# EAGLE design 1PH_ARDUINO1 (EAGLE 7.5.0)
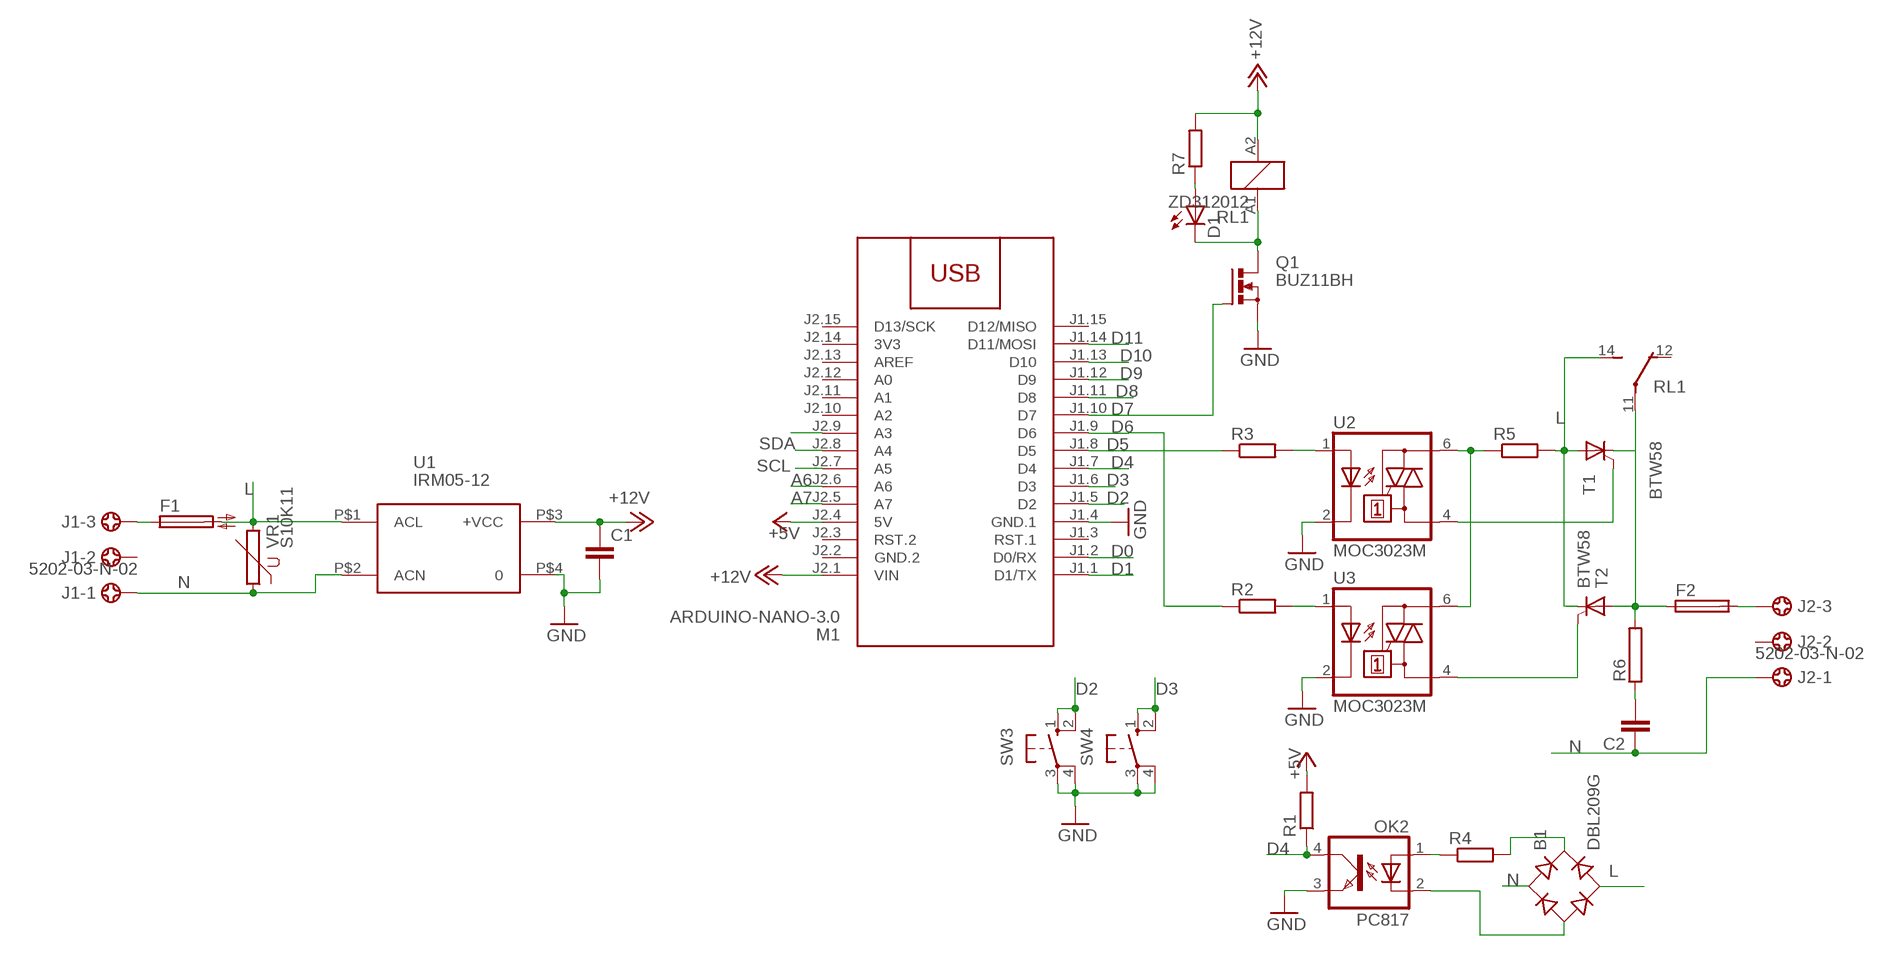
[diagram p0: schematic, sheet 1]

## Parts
B1  DBL209G  [DB]
C1  C-EUC1206  [C1206]
C2  C-EU150-084X183  [C150-084X183]
D1  LED5MM  [LED5MM]
F1  SH22,5A  [SH22,5A]
F2  SH22,5A  [SH22,5A]
J1  5202-03-N-02  [5202-03-N-02]
J2  5202-03-N-02  [5202-03-N-02]
M1  ARDUINO-NANO-3.0  [ARDUINO-NANO-3.0]
OK2  PC817  [DIL04]
Q1  BUZ11BH  [TO220BH]
R1  R-EU_R1206  [R1206]
R2  R-EU_R1206  [R1206]
R3  R-EU_R1206  [R1206]
R4  R-EU_R1206  [R1206]
R5  R-EU_R1206  [R1206]
R6  RAC07  [AC07]
R7  R-EU_R1206  [R1206]
RL1  ZD312012  [ZD1]
SW3  10-XX  [B3F-10XX]
SW4  10-XX  [B3F-10XX]
T1  BTW58  [TO220CS]
T2  BTW58  [TO220CS]
U1  IRM05-12  [IRM05-12]
U2  MOC3023M  [DIL06]
U3  MOC3023M  [DIL06]
VR1  S10K11  [S10K11]

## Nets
+5V: M1.J2.4(5V) R1.2
+12V: C1.1 M1.J2.1(VIN) R7.2 RL1.A2 U1.P$3(+VCC)
A3: M1.J2.9(A3)
A6: M1.J2.6(A6)
A7: M1.J2.5(A7)
D0: M1.J1.2(D0/RX)
D1: M1.J1.1(D1/TX)
D2: M1.J1.5(D2) SW3.1(S) SW3.2(S1)
D3: M1.J1.6(D3) SW4.1(S) SW4.2(S1)
D4: M1.J1.7(D4) OK2.4(COL) R1.1
D5: M1.J1.8(D5) R3.1
D6: M1.J1.9(D6) R2.1
D7: M1.J1.10(D7) Q1.G
D8: M1.J1.11(D8)
D9: M1.J1.12(D9)
D10: M1.J1.13(D10)
D11: M1.J1.14(D11/MOSI)
GND: C1.2 M1.J1.4(GND.1) OK2.3(EMIT) Q1.S SW3.3(P) SW3.4(P1) SW4.3(P) SW4.4(P1) U1.P$4 U2.2(C) U3.2(C)
L: B1.AC2 F1.2 R5.2 RL1.14(2:S) T1.A T2.C U1.P$1(ACL) VR1.2
N: B1.AC1 C2.1 J1.1 J2.1 U1.P$2(ACN) VR1.1
N$1: T2.G U3.4(A1)
N$2: R3.2 U2.1(A)
N$3: R2.2 U3.1(A)
N$4: R5.1 U2.6(A2) U3.6(A2)
N$5: B1.+ R4.2
N$6: OK2.1(A) R4.1
N$7: B1.- OK2.2(C)
N$8: F1.1 J1.3
N$9: T1.G U2.4(A1)
N$11: F2.1 R6.2 RL1.11(2:P) T1.C T2.A
N$12: D1.K(C) Q1.D RL1.A1
N$13: C2.2 R6.1
N$14: F2.2 J2.3
N$17: D1.A R7.1
SCL: M1.J2.7(A5)
SDA: M1.J2.8(A4)
Unconnected: J1.2 J2.2 M1.J1.3(RST.1) M1.J1.15(D12/MISO) M1.J2.3(RST.2) M1.J2.10(A2) M1.J2.11(A1) M1.J2.12(A0) M1.J2.13(AREF) M1.J2.15(D13/SCK) RL1.12(2:O)

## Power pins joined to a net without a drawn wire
3V3: M1.J2.14(3V3)
GND.2: M1.J2.2(GND.2)

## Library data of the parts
B1 = rectifier:DB?*G: Single Phase 1.0 AMP Glass Passivated Bridge Rectifier Taiwan Semiconductor Co.,Ltd. - TSC Source: http://www.taiwansemi.com/TSCbig5/ezcatfiles/cust/img/img/db101g.pdf http://www.ts.com.tw/db/pictures/modules/PDT/PDT060207001/DBLS201G.pdf
C1 C2 = rcl:C-EU: CAPACITOR, European symbol
D1 = led:LED: LED
F1 F2 = fuse:SH22,5A: FUSE HOLDER; MPN: 0031.7701.11; OC_FARNELL: unknown; OC_NEWARK: 04F1224
J1 J2 = con-ebyelectro:5202-03-N-02: Barrier Blocks Sreies 5202 Source: http://www.ebyelectro.com/PDF/5202-XX-N-02.pdf; OC_FARNELL: unknown; OC_NEWARK: unknown
M1 = diy-modules:ARDUINO-NANO-3.0: Arduino Nano 3.0 and compatible devices More details available here: https://www.arduino.cc/en/Main/ArduinoBoardNano Click here to find device on ebay.com
OK2 = optocoupler:PC817: SHARP OPTO COUPLER; MPN: PC817X4J000F; OC_FARNELL: 9707727; OC_NEWARK: 97K7059
Q1 = transistor-power:BUZ11: N-CHANNEL MOS FET
R1-R5 R7 = rcl:R-EU_: RESISTOR, European symbol
R6 = resistor-power:R: Power Resitor; OC_FARNELL: unknown; OC_NEWARK: unknown
RL1 = relay:ZD?1*: Power Relay SCHRACK 1 pole 30 A Source: http://www.schrack.com/.. 5848.pdf; OC_FARNELL: unknown; OC_NEWARK: unknown
SW3 SW4 = switch-omron:10-XX: OMRON SWITCH; MPN: B3F-1000; OC_FARNELL: 176432; OC_NEWARK: 36M3542
T1 T2 = triac:BTW58: THYRISTOR
U1 = acdc:IRM05-12
U2 U3 = optocoupler:MOC30*M: RANDOM-PHASE OPTOISOLATORS TRIAC DRIVER OUTPUT Source: http://www.fairchildsemi.com MOC3020-M.pdf; MF: FAIRCHILD SEMICONDUCTOR; MPN: MOC3023-M; OC_FARNELL: 1021367; OC_NEWARK: 72K8896
VR1 = varistor:S10K11: VARISTOR

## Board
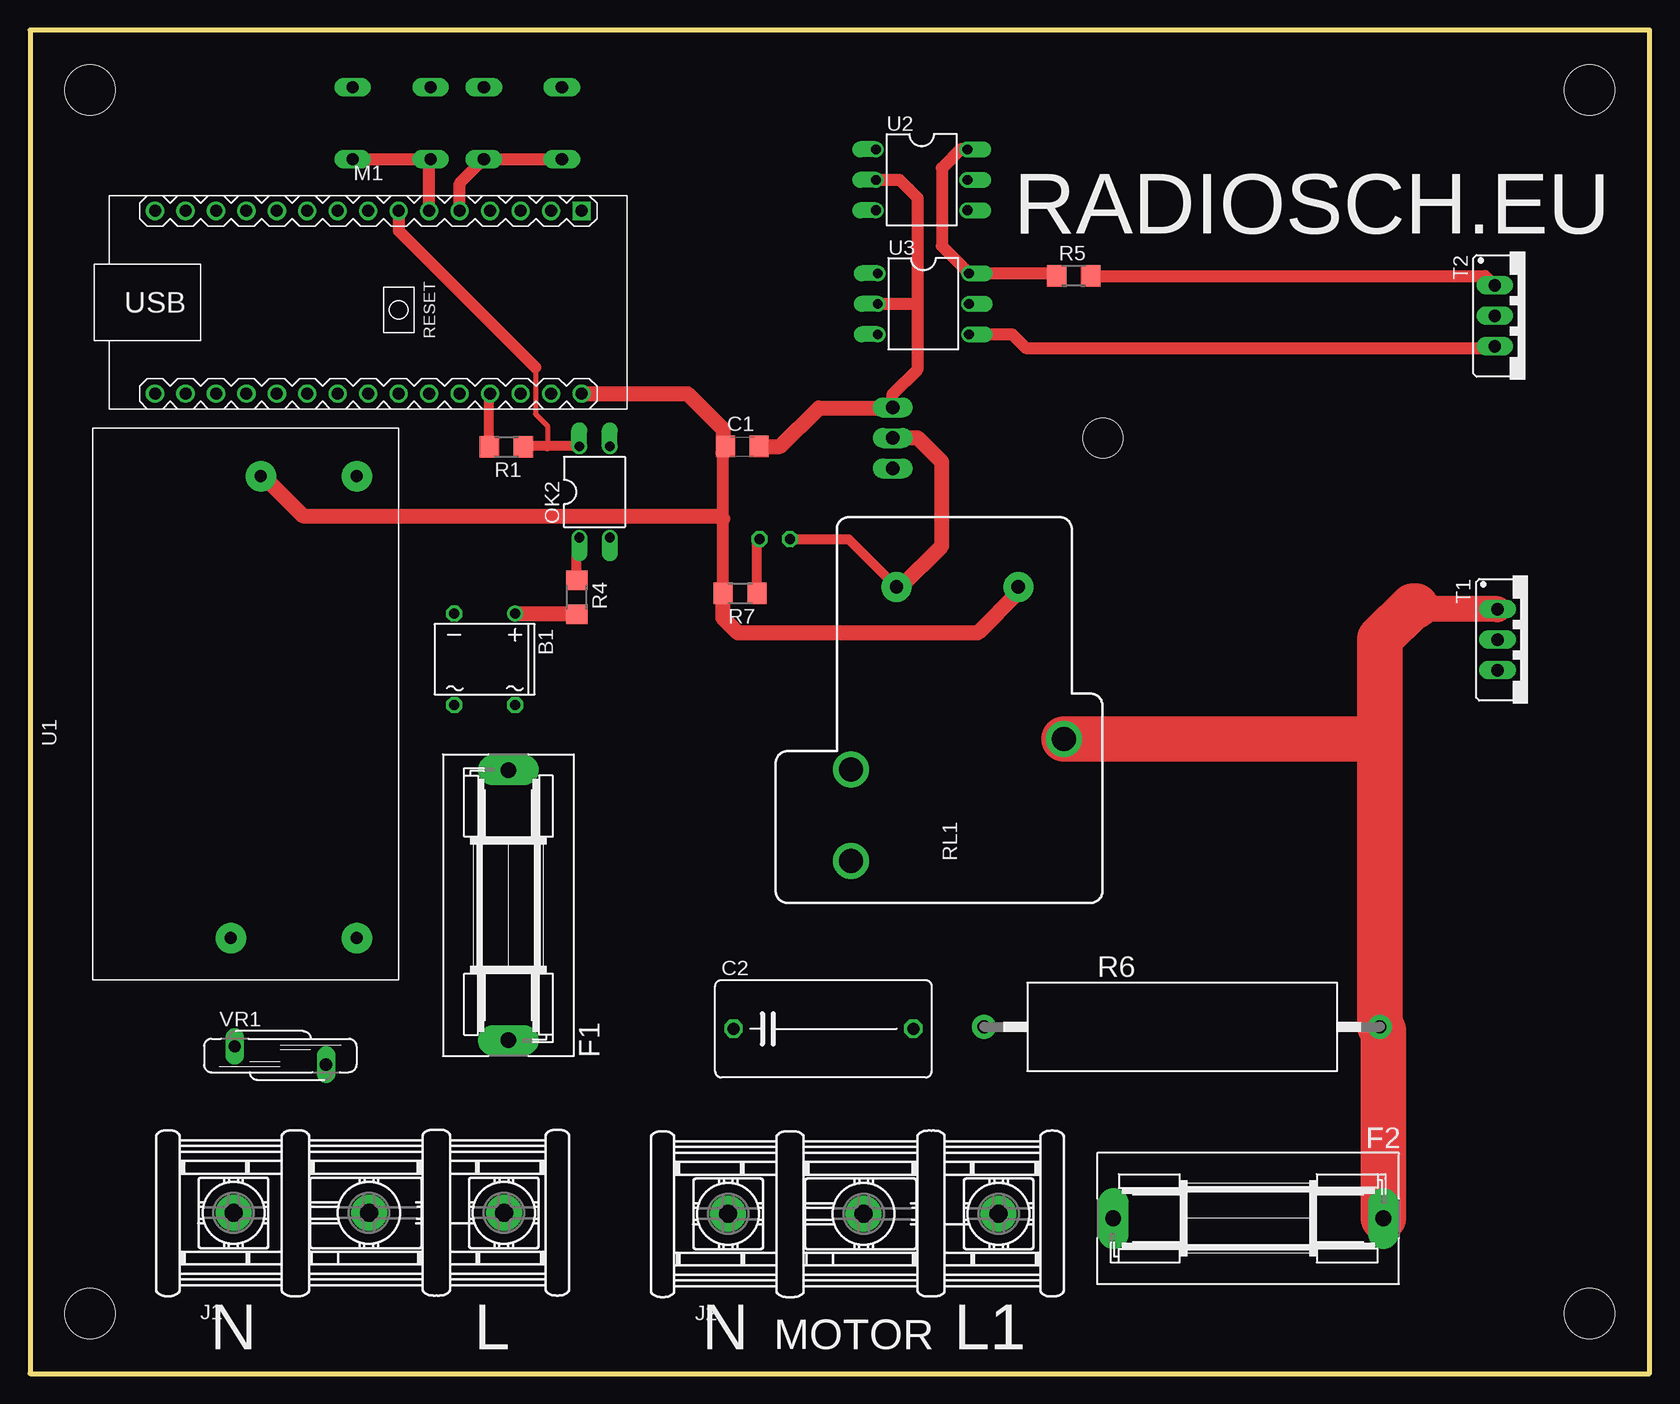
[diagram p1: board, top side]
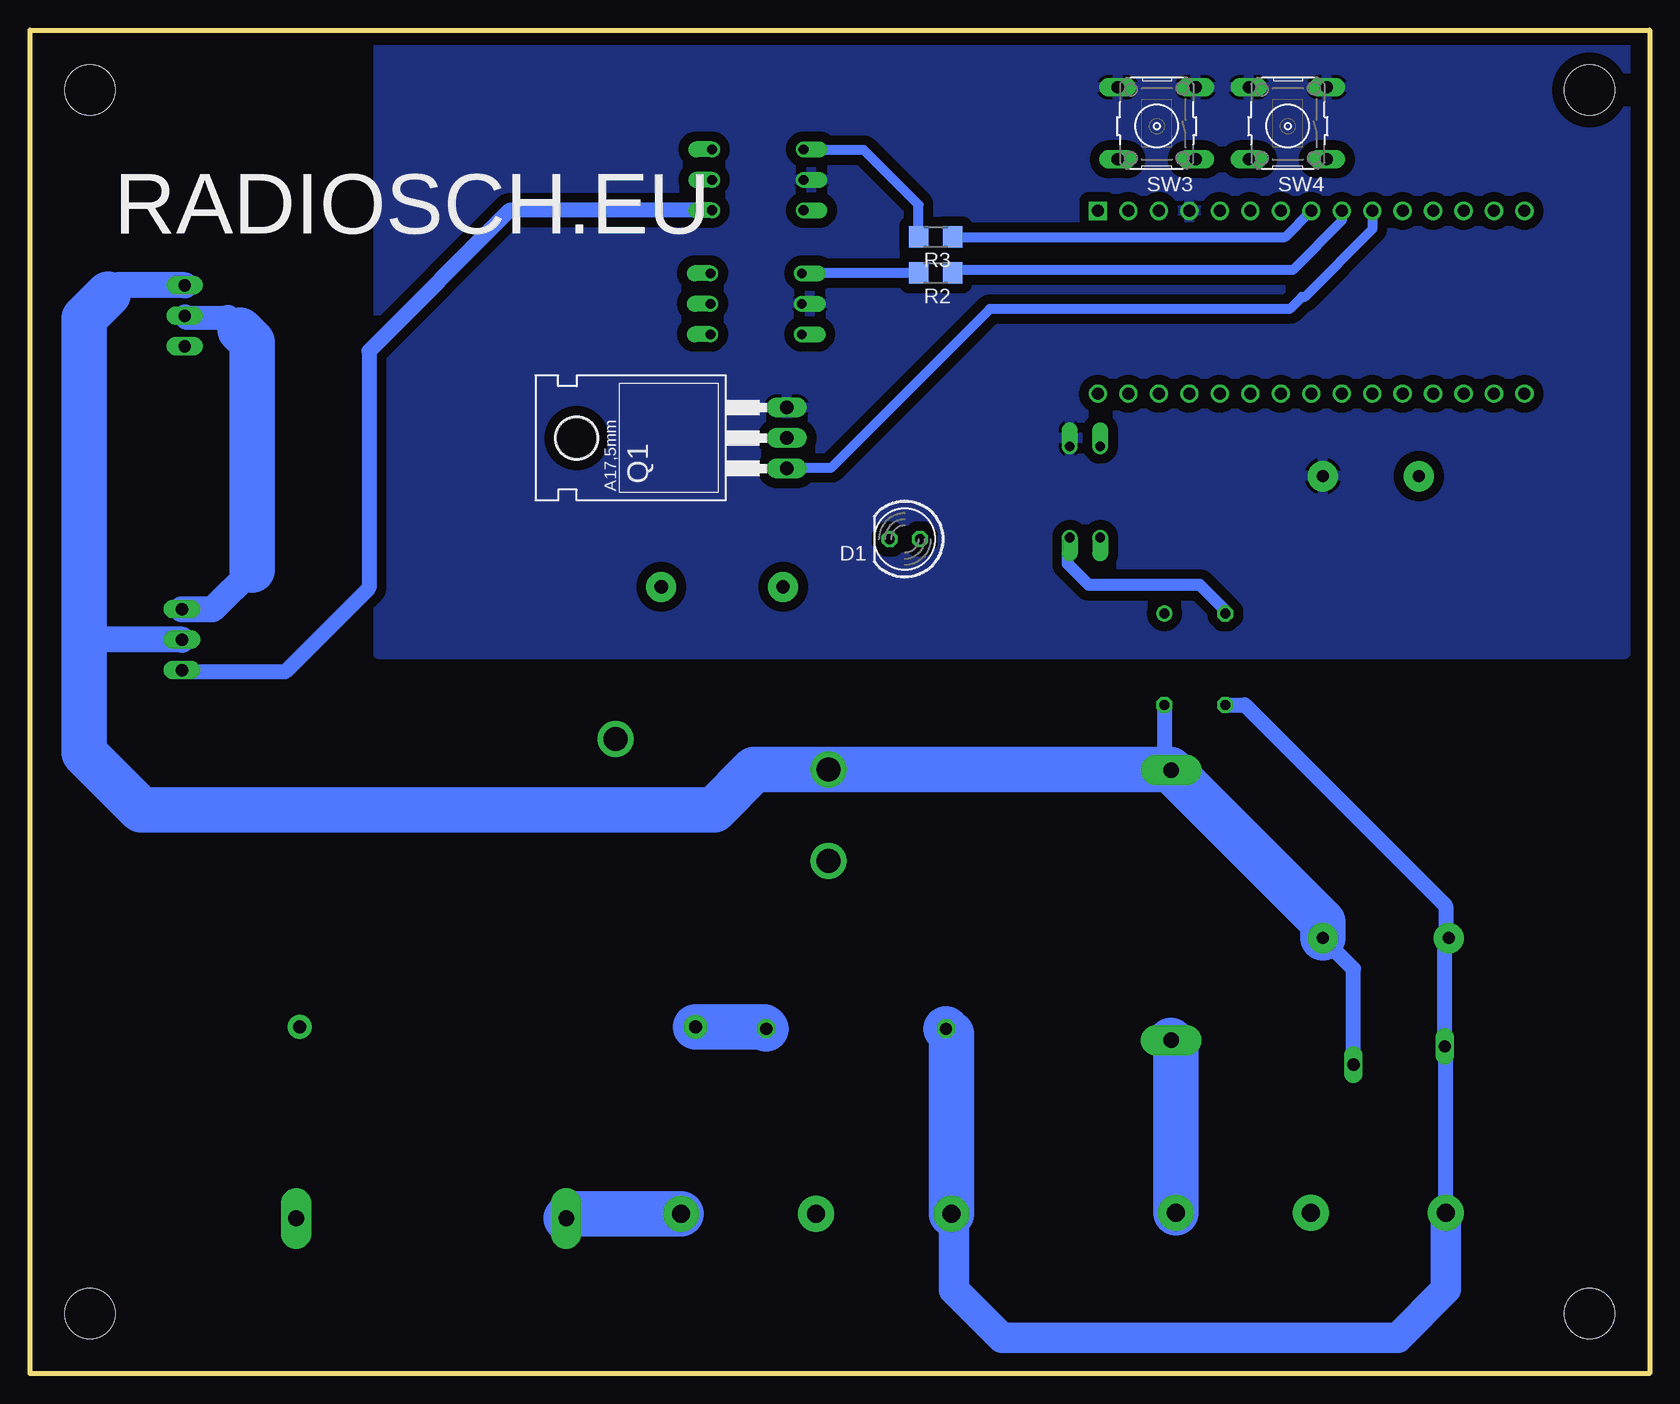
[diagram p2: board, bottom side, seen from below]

Size 135 x 112 mm. Coordinates in mm from the lower left corner, seen from the top.
Outline: 0,0 135,0 135,112 0,112 0,0
Copper layers (1*16): Top 0.035mm / dielectric 1.5mm / Bottom 0.035mm
Design rules "default": minimum track width 10mil, minimum drill 24mil, track to track 8mil, track to pad 8mil, pad to pad 8mil, via to via 8mil, smd to smd 8mil, copper to edge 40mil, drill to drill 8mil, minimum pad ring 10mil, minimum via ring 8mil, stop-mask expansion 4mil, vias tented up to drill 0mil, thermal gap 10mil
Holes 4.2 mm at 5,107 130,107 130,5 5,5

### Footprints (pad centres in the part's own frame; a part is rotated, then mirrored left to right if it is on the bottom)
DB = drill 0.813: + -2.54,-3.81 | drill 0.813 octagon: - 2.54,-3.81; AC1 2.54,3.81; AC2 -2.54,3.81
C1206 = smd 1.6 x 1.8: 1 -1.4,0; 2 1.4,0
C150-084X183 = drill 1.016 octagon: 1 -7.493,0; 2 7.493,0
LED5MM = drill 0.813 octagon: A -1.27,0; K 1.27,0
SH22,5A = drill 1.321 pad 2.54 long: 1 -11.252,0; 2 11.252,0
5202-03-N-02 = drill 1.5 pad 3: 1 -9.29,0; 2 2,0; 3 13.25,0
ARDUINO-NANO-3.0 = drill 1 square: J1.1 17.78,7.62 | drill 1: J1.2 15.24,7.62; J1.3 12.7,7.62; J1.4 10.16,7.62; J1.5 7.62,7.62; J1.6 5.08,7.62; J1.7 2.54,7.62; J1.8 0,7.62; J1.9 -2.54,7.62; J1.10 -5.08,7.62; J1.11 -7.62,7.62; J1.12 -10.16,7.62; J1.13 -12.7,7.62; J1.14 -15.24,7.62; J1.15 -17.78,7.62; J2.1 17.78,-7.62; J2.2 15.24,-7.62; J2.3 12.7,-7.62; J2.4 10.16,-7.62; J2.5 7.62,-7.62; J2.6 5.08,-7.62; J2.7 2.54,-7.62; J2.8 0,-7.62; J2.9 -2.54,-7.62; J2.10 -5.08,-7.62; J2.11 -7.62,-7.62; J2.12 -10.16,-7.62; J2.13 -12.7,-7.62; J2.14 -15.24,-7.62; J2.15 -17.78,-7.62
DIL04 = drill 0.813 offset: 1 -1.27,-3.81; 2 1.27,-3.81; 3 1.27,3.81; 4 -1.27,3.81
TO220BH = drill 1.118 long: D 0,-6.35; G -2.54,-6.35; S 2.54,-6.35 | hole 3.302: 0,11.176
R1206 = smd 1.6 x 1.803: 1 -1.422,0; 2 1.422,0
AC07 = drill 1.1 pad 2: 1 -16.5,0; 2 16.5,0
ZD1 = drill 2 pad 2.5: 11 -2.54,-8.88; 12 -12.7,8.88; 14 -5.08,8.88 | drill 1.1 pad 2.5: A1 10.16,5.08; A2 10.16,-5.08
B3F-10XX = drill 1.016 long: 1 -3.251,2.761; 2 3.251,2.761; 3 -3.251,-3.261; 4 3.251,-3.261
TO220CS = drill 1.016 long: A 0,-2.54; C -2.54,-2.54; G 2.54,-2.54
IRM05-12 = drill 1 pad 2.54: P$1 3.5,3.5; P$2 3.5,14; P$3 42,11.5; P$4 42,3.5
DIL06 = drill 0.813 offset: 1 -2.54,-3.81; 2 0,-3.81; 3 2.54,-3.81; 4 2.54,3.81; 5 0,3.81; 6 -2.54,3.81
S10K11 = drill 1.016 long: 1 -0.762,-3.81; 2 0.762,3.81

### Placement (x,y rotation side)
B1  37.9,59.54 180 top
C1  59.37,77.28 0 top
C2  66.14,28.74 0 top
D1  62.08,69.56 180 bottom
F1  39.88,39.04 90 top
F2  101.55,12.93 180 top
J1  26.25,13.39 0 top
J2  67.49,13.31 0 top
M1  28.2,89.3 0 top
OK2  47.06,73.49 0 top
Q1  78.26,77.99 90 bottom
R1  39.71,77.26 180 top
R2  59.5,91.75 180 bottom
R3  59.5,94.75 180 bottom
R4  45.57,64.71 270 top
R5  87,91.5 0 top
R6  96.03,28.9 0 top
R7  59.19,65.04 180 top
RL1  77.3,55.42 90 top
SW3  41.08,103.98 180 bottom
SW4  30.15,103.98 180 bottom
T1  124.87,61.17 270 top
T2  124.64,88.17 270 top
U1  30.73,32.81 90 top
U2  74.33,99.51 270 top
U3  74.47,89.17 270 top
VR1  20.86,26.51 270 top

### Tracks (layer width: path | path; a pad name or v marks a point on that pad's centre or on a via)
+5V
  Top 0.813: R1.2 38.29,81.61 M1.J2.4
+12V
  Top 1.016: R7.2 57.77,71.25 57.77,76.75 57.77,77.08 C1.1
  Top 1.27: U1.P$3 19.44,74.81 22.75,71.5 57.52,71.5 57.77,71.25 | M1.J2.1 54.82,81.68 57.75,78.75 57.75,76.77 57.77,76.75 | RL1.A2 82.38,65.13 79,61.75 59,61.75 57.75,63 57.75,65.02 R7.2
D2
  Top 1.016: M1.J1.5 35.82,99.21 SW3.1 SW3.2
D3
  Top 1.016: M1.J1.6 33.28,101.1 SW4.2 SW4.1
D4
  Top 0.406: 42.12,83.88 42.12,80 43.12,79 43.12,77.3
  Top 0.813: OK2.4 43.12,77.3 41.17,77.3 R1.1
  Top 1.016: M1.J1.7 30.74,95.26 42.12,83.88
D5
  Bottom 0.813: R3.1 30.37,94.75 M1.J1.8
D6
  Bottom 0.813: M1.J1.9 25.66,96.09 29.75,92 57.83,92 R2.1
D7
  Bottom 0.813: M1.J1.10 23.12,95.38 28.75,89.75 29,89.75 30,88.75 55,88.75 68.25,75.5 71.86,75.5 Q1.G
GND
  Top 1.016: Q1.S 71.91,81.66 74,83.75 74,89 | 74,89 74,98 72.5,99.5 U2.2 | U3.2 73.83,89.17 74,89
  Top 1.27: C1.2 62.53,77.28 65.75,80.5 71.88,80.5 Q1.S
  pour Bottom (isolate 0.813): 2,111 106,111 106,60 2,60
L
  Top 1.016: R5.2 121.31,91.5 T2.C
  Bottom 1.27: VR1.2 24.67,33.75 U1.P$1 | B1.AC2 40.44,50.85 F1.2
  Bottom 2.184: T2.C 127.79,90.71 128.5,90 | T1.A 130.25,61.17 130.33,61.17 130.5,61
  Bottom 3.81: U1.P$1 27.23,37.64 F1.2 39.93,50.34 RL1.14 74.66,50.34 78,47 125.75,47 130.5,51.75 130.5,60.92 130.25,61.17 | 130.5,61 130.5,88 128.5,90
N
  Bottom 1.27: J1.1 16.96,27.18 VR1.1 17.05,35.99 U1.P$2 17,36.58 17,39 33.73,55.73 B1.AC1
  Bottom 2.54: J1.1 16.96,7.04 21,3 54,3 58,7 58,13.11 J2.1
  Bottom 3.81: J2.1 58.2,28.29 C2.1
N$1
  Top 1.016: U3.4 81.87,86.63 83,85.5 121.97,85.5 T2.G
N$2
  Bottom 0.813: R3.2 60.92,97.42 65.5,102 70.47,102 U2.1
N$3
  Bottom 0.813: R2.2 70.62,91.75 U3.1
N$4
  Top 1.016: R5.1 85.37,91.71 U3.6 76,93.99 76,100.5 77.55,102.05 U2.6
N$5
  Top 1.27: B1.+ 45.51,63.35 R4.2
N$6
  Top 0.813: R4.1 45.57,69.46 OK2.1
N$7
  Bottom 1.016: B1.- 35.36,63.61 37.5,65.75 46.75,65.75 48.5,67.5 48.5,69.51 OK2.2
N$8
  Bottom 3.81: J1.3 39.5,27.41 F1.1
N$9
  Bottom 1.27: U2.4 95.03,96.97 106.75,85.25 106.75,65.5 113.75,58.5 122.2,58.5 T1.G
N$11
  Top 2.184: T1.C 115.79,63.71 115.5,64
  Top 3.81: 115.5,64 115.25,64 112.53,61.28 112.53,53 | F2.1 112.8,28.63 R6.2 112.53,53 | RL1.11 112.41,52.88 112.53,53
  Bottom 1.93: 121.93,88 T2.A
  Bottom 2: 118.5,88 121.93,88
  Bottom 2.184: T1.C 119.79,63.71 116.5,67 | 117.5,87 118.5,88
  Bottom 3.81: 116.5,67 116.5,86 117.5,87
N$12
  Top 0.813: D1.K 68.24,69.56 RL1.A1
  Top 1.27: RL1.A1 72.58,65.58 76,69 76,76 74,78 Q1.D
N$13
  Bottom 3.81: R6.1 73.79,28.9 C2.2
N$14
  Bottom 3.81: J2.3 89.92,13.31 F2.2
N$17
  Top 0.813: R7.1 60.61,69.36 D1.A

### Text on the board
tPlace: RADIOSCH.EU | N | L | N | MOTOR | L1
bPlace: RADIOSCH.EU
